PROGRAM MAIN
VAR
	drive:		DriveTyp;
	down:		DownTyp;
	up:			UpTyp;
END_VAR

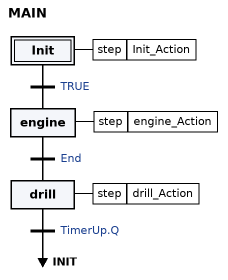
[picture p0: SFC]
INITIAL_STEP Init:
    Init_Action(N);  // step action
END_STEP
TRANSITION FROM Init TO engine
    := TRUE;
END_TRANSITION
STEP engine:
    engine_Action(N);  // step action
END_STEP
TRANSITION FROM engine TO drill
    := End;
END_TRANSITION
STEP drill:
    drill_Action(N);  // step action
END_STEP
TRANSITION FROM drill TO INIT
    := TimerUp.Q;
END_TRANSITION

ACTION DevDown_Action:
// NETWORK 1
// instruction list
CAL     Down
END_ACTION

ACTION DevInit_Action:
engine.x := FALSE;
count := count + 1;
END_ACTION

ACTION DevUp_Action:
// NETWORK 1
// instruction list
CAL     UP
END_ACTION

ACTION drill_Action:
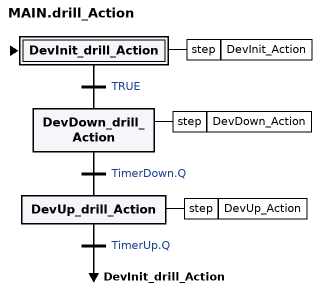
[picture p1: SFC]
INITIAL_STEP DevInit_drill_Action:
    DevInit_Action(N);  // step action
END_STEP
TRANSITION FROM DevInit_drill_Action TO DevDown_drill_Action
    := TRUE;
END_TRANSITION
STEP DevDown_drill_Action:
    DevDown_Action(N);  // step action
END_STEP
TRANSITION FROM DevDown_drill_Action TO DevUp_drill_Action
    := TimerDown.Q;
END_TRANSITION
STEP DevUp_drill_Action:
    DevUp_Action(N);  // step action
END_STEP
TRANSITION FROM DevUp_drill_Action TO DevInit_drill_Action
    := TimerUp.Q;
END_TRANSITION
END_ACTION

TRANSITION End:
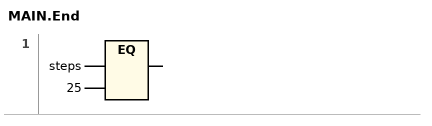
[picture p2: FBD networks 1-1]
// NETWORK 1
(* steps = 25; result not used *)
END_TRANSITION

ACTION engine_Action:
drive();
END_ACTION

ACTION Init_Action:
// NETWORK 1
//  initialize Variables
// instruction list
LD      TRUE
R       engine.x
R       deviceUp
R       deviceDown
LD      0
ST      steps
LD      TRUE
R       timerDown.IN
CAL     timerDown
LD      TRUE
R       timerUp.IN
CAL     timerUp
END_ACTION

END_PROGRAM
